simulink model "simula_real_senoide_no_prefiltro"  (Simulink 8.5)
settings: Solver=ode45  StartTime=0.0  StopTime=tf  FixedStep=dt  RelTol=1e-6
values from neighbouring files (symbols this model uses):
  Areal = [zeros(n2,n2) eye(n2); -Pinv*R -Pinv*Q]    [mod_estados_real.m]
  Breal = [zeros(n2,1); Pinv*U]    [mod_estados_real.m]
  Creal = zeros(1,2*n2)    [mod_estados_real.m]
  denF = [1 qsi2wn wn2]    [princi_JL_incerto_prefilt_2a_ordem.m]
  denK = [1/6 1]    [princi_JL_incerto_prefilt_2a_ordem.m]
  Dreal = 0    [mod_estados_real.m]
  numF = [wn2]    [princi_JL_incerto_prefilt_2a_ordem.m]
  numK = 2.5    [princi_JL_incerto_prefilt_2a_ordem.m]
  w0_pre_filt = wF    (= 0.36)    [princi_JL_incerto_prefilt_2a_ordem.m]

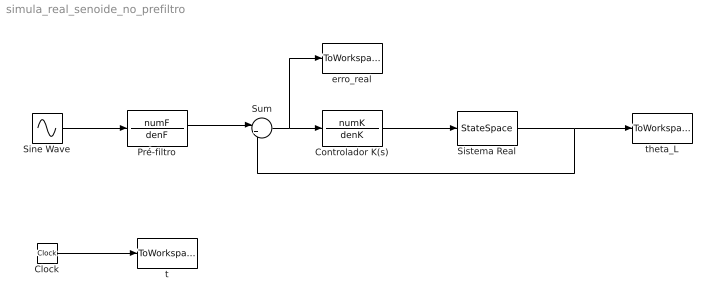
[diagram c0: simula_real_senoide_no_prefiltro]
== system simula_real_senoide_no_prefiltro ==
  Clock : Clock
  Controlador K(s) : TransferFcn  Numerator=numK  Denominator=denK
  Pré-filtro : TransferFcn  Numerator=numF  Denominator=denF
  Sine Wave : Sin  Frequency=w0_pre_filt  SampleTime=0
  Sistema Real : StateSpace  A=Areal  B=Breal  C=Creal  D=Dreal  X0=0
  Sum : Sum  Inputs=|+-
  erro_real : ToWorkspace  VariableName=erro_real  SampleTime=-1
  t : ToWorkspace  VariableName=t  SampleTime=-1
  theta_L : ToWorkspace  VariableName=theta_L_real  SampleTime=-1
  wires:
  Sum/1 -> erro_real/1, Controlador K(s)/1
  Pré-filtro/1 -> Sum/1
  Clock/1 -> t/1
  Controlador K(s)/1 -> Sistema Real/1
  Sistema Real/1 -> Sum/2, theta_L/1
  Sine Wave/1 -> Pré-filtro/1
